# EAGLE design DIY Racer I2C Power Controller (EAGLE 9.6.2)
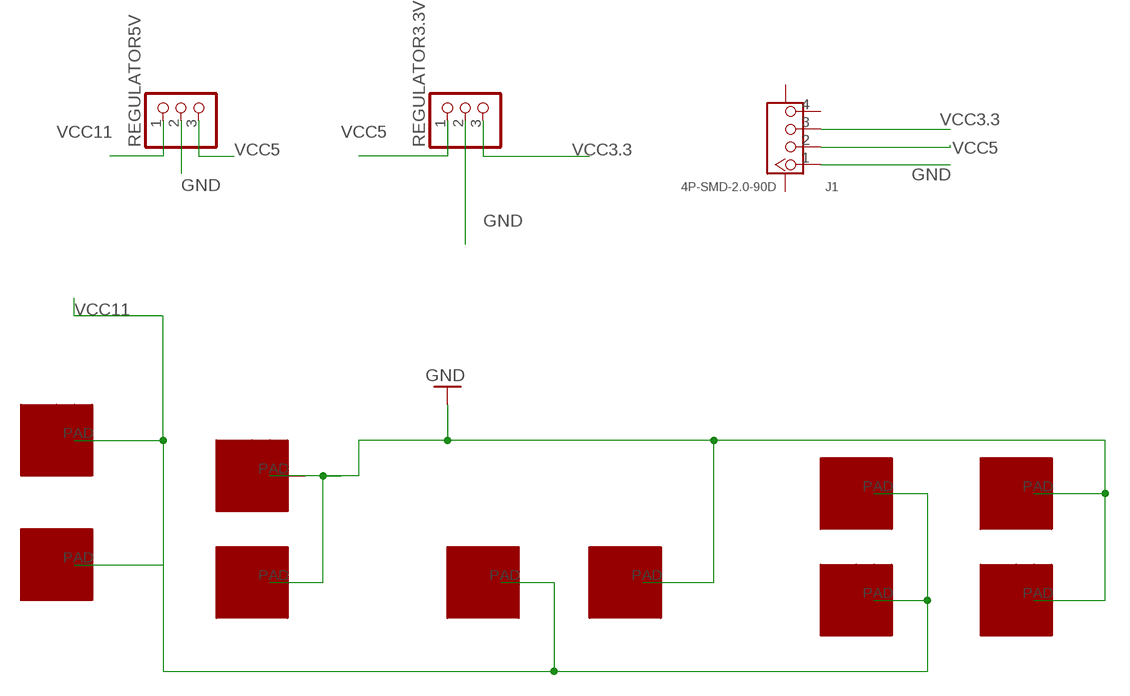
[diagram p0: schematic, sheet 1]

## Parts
J1  4P-SMD-2.0-90D  GROVE-CONNECTOR-SMD-90D(4+2P-2.0)  [HW4-SMD-2.0-90D]
REGULATOR3.3V  PINHD-1X03_2.54-SMD  [1X03SMD]
REGULATOR5V  PINHD-1X03_2.54-SMD  [1X03SMD]
U$4  MYPAD  [MYPAD]
U$5  MYPAD  [MYPAD]
U$6  MYPAD  [MYPAD]
U$7  MYPAD  [MYPAD]
U$8  MYPAD  [MYPAD]
U$9  MYPAD  [MYPAD]
U$10  MYPAD  [MYPAD]
U$11  MYPAD  [MYPAD]
U$12  MYPAD  [MYPAD]
U$13  MYPAD  [MYPAD]

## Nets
GND: J1.1 REGULATOR3.3V.2 REGULATOR5V.2 U$6.PAD(VCC) U$7.PAD(VCC) U$10.PAD(VCC) U$11.PAD(VCC) U$13.PAD(VCC)
VCC3.3: J1.3 REGULATOR3.3V.3
VCC5: J1.2 REGULATOR3.3V.1 REGULATOR5V.3
VCC11: REGULATOR5V.1 U$4.PAD(VCC) U$5.PAD(VCC) U$8.PAD(VCC) U$9.PAD(VCC) U$12.PAD(VCC)
Unconnected: J1.4 J1.SS1 J1.SS2

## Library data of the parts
J1 = OPL_Connector:GROVE-CONNECTOR-SMD-90D(4+2P-2.0): 320110032
REGULATOR3.3V REGULATOR5V = pinhead-2:PINHD-1X03: PIN HEADER
U$4-U$13 = custom:MYPAD: ESC and Battery PAD

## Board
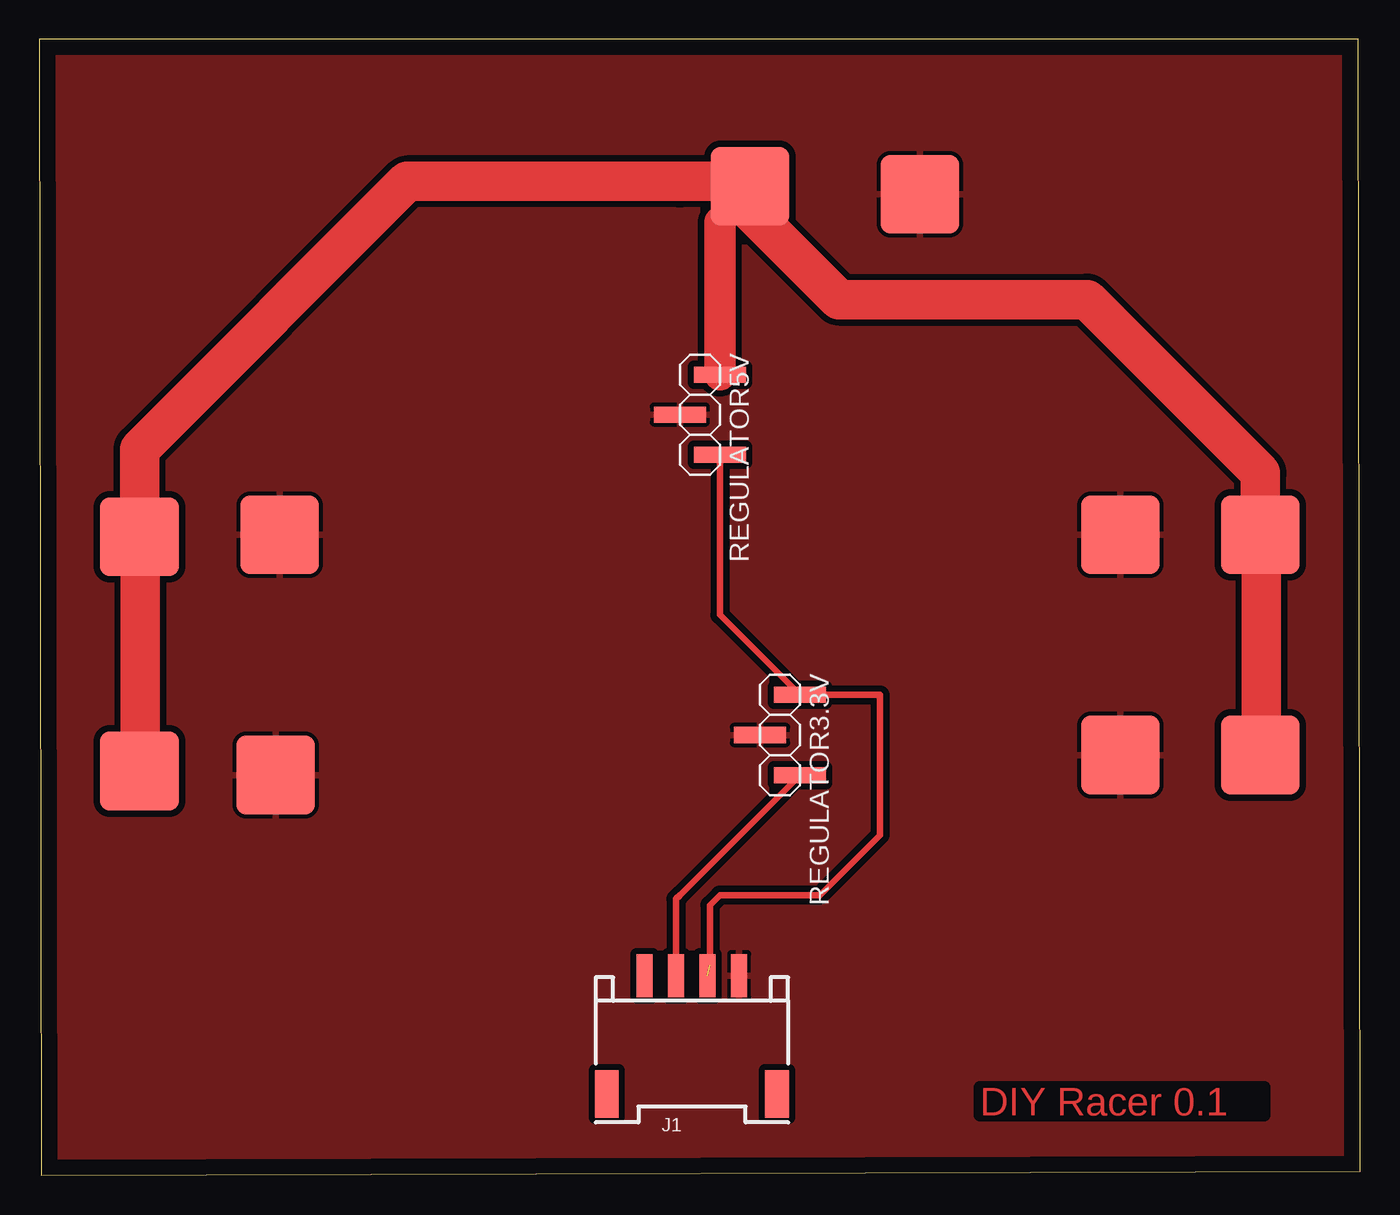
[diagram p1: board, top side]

Size 83.8 x 72.06 mm. Coordinates in mm from the lower left corner, seen from the top.
Outline: 0.13,0 83.8,0.25 83.67,72.06 0,72.06 0.13,0
Copper layers (1*16): Top 0.035mm / dielectric 1.5mm / Bottom 0.035mm
Design rules "default *": minimum track width 0.4mm, minimum drill 0.35mm, track to track 0.4mm, track to pad 0.4mm, pad to pad 0.4mm, via to via 4mm, smd to smd 0.4mm, copper to edge 40mil, drill to drill 6mil, minimum pad ring 10mil, minimum via ring 8mil, stop-mask expansion 4mil, vias tented up to drill 0mil, thermal gap 10mil

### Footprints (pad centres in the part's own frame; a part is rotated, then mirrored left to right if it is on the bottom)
HW4-SMD-2.0-90D = smd 1.01 x 2.74: 1 -3,-0.1; 2 -1,-0.1; 3 1,-0.1; 4 3,-0.1 | smd 1.5 x 3: SS1 -5.4,7.4; SS2 5.4,7.4
1X03SMD = smd 1.016 x 3.302: 1 -1.27,1.27; 2 1.27,-1.27; 3 3.81,1.27
MYPAD = smd 5 x 5: PAD 0,0

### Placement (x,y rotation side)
J1  41.4,12.57 180 top
REGULATOR3.3V  46.99,29.21 270 top
REGULATOR5V  41.91,49.53 270 top
U$4  45.09,62.74 0 top
U$5  6.35,40.51 0 top
U$6  14.99,25.4 0 top
U$7  15.24,40.64 0 top
U$8  6.35,25.65 0 top
U$9  77.47,40.64 0 top
U$10  55.88,62.23 0 top
U$11  68.58,40.64 0 top
U$12  77.47,26.67 0 top
U$13  68.58,26.67 0 top

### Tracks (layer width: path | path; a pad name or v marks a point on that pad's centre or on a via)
GND
  Top 0.4: 16.51,40.64 14.99,39.12
  pour Top: 0,72.39 114.3,72.39 114.3,-13.97 0,-13.97
VCC3.3
  Top 0.4: REGULATOR3.3V.3 40.64,17.78 40.4,17.54 | 40.4,17.54 40.39,17.53 | 40.4,17.54 J1.3
VCC5  (1 unrouted)
  Top 0.4: 43.2,43.37 43.2,45.7 REGULATOR5V.3 43.18,35.56 REGULATOR3.3V.1 | REGULATOR3.3V.1 49.53,30.48 | REGULATOR3.3V.1 53.34,30.48 53.34,21.59 49.53,17.78 43.18,17.78 42.55,17.14 42.55,13.34
VCC11
  Top 0.4: 43.2,50.9 REGULATOR5V.1 | 77.52,26.69 U$12.PAD | 77.52,40.57 U$9.PAD | 6.4,25.7 U$8.PAD | 6.4,40.5 U$5.PAD | 44.8,61.37 44.8,62.5 U$4.PAD | U$4.PAD 45.09,61.2 | 40.64,63.06 41.08,63.5 44.45,63.5 44.45,61.72 43.18,60.45 43.18,60.83 U$4.PAD
  Top 2: REGULATOR5V.1 43.18,60.45
  Top 2.5: 77.52,40.57 77.52,26.69 | 6.4,40.5 6.4,25.7 | U$5.PAD 6.35,46.07 23.34,63.06 40.64,63.06 43.2,63.06 | U$9.PAD 77.47,44.57 66.48,55.56 50.73,55.56 45.09,61.2

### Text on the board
Top: DIY Racer 0.1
